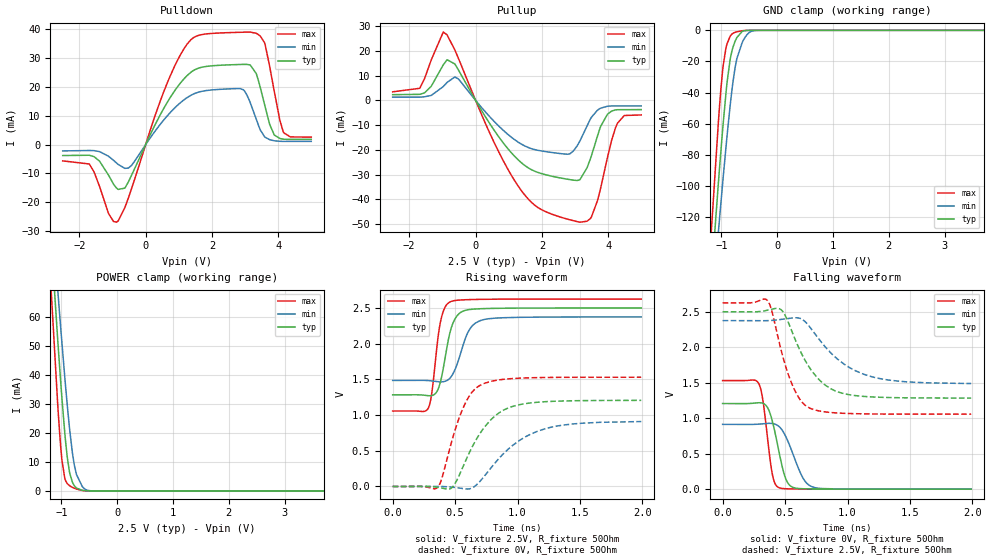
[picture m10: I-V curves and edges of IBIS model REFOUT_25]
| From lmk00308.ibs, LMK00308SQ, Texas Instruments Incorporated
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|   Model REFOUT_25
[Model]   REFOUT_25
Model_type   Output
Polarity   Non-Inverting
Rref =   50.0000
Vref =   1.25
Vmeas =   1.25
|   typ   min   max
C_comp   0.4681pF   0.4606pF   0.4681pF
|Output in low   Nom   Weak   Strong
|C_Comp   0.4681pF   0.4606pF   0.4681pF
|Output in High   Nom   Strong   Weak
|C_Comp High   0.4470pF   0.4470pF   0.4539pF
|Output in Hi-Z   Nom   Strong   Weak
|C_Comp   0.5714pF   0.5375pF   0.5943pF
[Voltage Range]   2.5   2.375   2.625
[Temperature Range]   45   125   -40
[Pullup Reference]   2.5   2.375   2.625
[Pulldown Reference]   0   0   0
[Power Clamp Reference]   2.5   2.375   2.625
[GND Clamp Reference]   0   0   0
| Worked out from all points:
|   slope of the pulldown table from 0 to 0.375 V, typ, clamps not added: 42 ohm
|   slope of the pullup table from 0 to 0.375 V, typ, clamps not added: 45.2 ohm
|   GND clamp passes 1 mA (typ) near -0.63 V on its own axis
|   POWER clamp passes 1 mA (typ) near -0.73 V on its own axis
|   falling waveform, V_fixture 0V, R_fixture 50Ohm: 20-80 % time 91.2ps typ, 127ps min, 64.1ps max; typ from 1.21 V to 0 V
|   rising waveform, V_fixture 2.5V, R_fixture 50Ohm: 20-80 % time 85.5ps typ, 110ps min, 65.7ps max; typ from 1.28 V to 2.5 V
|   rising waveform, V_fixture 0V, R_fixture 50Ohm: 20-80 % time 250ps typ, 348ps min, 176ps max; typ from 0 V to 1.21 V
|   falling waveform, V_fixture 2.5V, R_fixture 50Ohm: 20-80 % time 234ps typ, 332ps min, 163ps max; typ from 2.5 V to 1.28 V
[Pulldown]
|   Voltage   I(typ)   I(min)   I(max)
-2.5V     -3.786mA   -2.179mA   -5.641mA
-1.698V   -3.679mA   -2.038mA   -6.725mA
-1.12V    -10.57mA   -4.022mA   -23.89mA
-827.5mV  -15.55mA   -6.873mA   -26.48mA
-422.5mV  -10.57mA   -7.175mA   -15.18mA
890mV     18.94mA    12.9mA     27.64mA
1.895V    27.24mA    18.87mA    38.51mA
2.945V    27.86mA    19.05mA    39.03mA
3.455V    19.87mA    5.117mA    37.69mA
3.875V    3.399mA    1.343mA    18.61mA
4.145V    1.907mA    1.124mA    4.528mA
4.992V    1.816mA    1.12mA     2.598mA
[GND Clamp]
|   Voltage   I(typ)   I(min)   I(max)
-2.5V     -850.7mA   -783.9mA   -946.5mA
-1.202V   -170.8mA   -193.7mA   -141.7mA
-1.052V   -97.92mA   -129.5mA   -58.7mA
-1.038V   -90.97mA   -123.2mA   -51.32mA
-970mV    -61.13mA   -95.72mA   -23.37mA
-917.5mV  -40.48mA   -75.29mA   -11.35mA
-842.5mV  -18.81mA   -48.55mA   -3.881mA
-790mV    -10.67mA   -32.74mA   -1.863mA
-722.5mV  -4.664mA   -18.24mA   -948.5uA
-625mV    -674.1uA   -7.739mA   -269.5uA
-415mV    -2.631uA   -208.5uA   -1.695uA
4.992V    0A         0A         0A
[Pullup]
|   Voltage   I(typ)   I(min)   I(max)
-2.5V     2.292mA    1.299mA    3.442mA
-1.683V   2.418mA    1.287mA    4.854mA
-970mV    14.41mA    5.628mA    27.54mA
-520mV    12.32mA    8.65mA     17.02mA
537.5mV   -11.63mA   -8.192mA   -16.39mA
1.363V    -24.97mA   -17.52mA   -36.09mA
2.78V     -31.85mA   -21.73mA   -47.97mA
3.147V    -31.96mA   -16.32mA   -49.17mA
3.493V    -22.32mA   -6.811mA   -47.02mA
3.973V    -5.672mA   -2.384mA   -23.2mA
4.28V     -3.776mA   -2.257mA   -9.165mA
4.992V    -3.74mA    -2.236mA   -5.891mA
[POWER Clamp]
|   Voltage   I(typ)   I(min)   I(max)
-2.5V     504.8mA    460mA      565.3mA
-1.21V    94.23mA    106.3mA    77.92mA
-1.06V    50.38mA    67.9mA     27.85mA
-992.5mV  32.36mA    51.45mA    10.86mA
-940mV    20.01mA    39.28mA    4.347mA
-895mV    11.57mA    29.52mA    2.526mA
-850mV    6.048mA    20.73mA    1.745mA
-797.5mV  2.773mA    12.35mA    1.177mA
-730mV    975.1uA    5.644mA    633.8uA
-625mV    202.7uA    1.451mA    147.7uA
-490mV    13.53uA    84.98uA    8.561uA
4.992V    0A         0A         0A
[Ramp]
R_load = 50
|   typ   min   max
dV/dt_r   0.729929/8.55058e-11   0.533736/1.09569e-10   0.940882/6.56837e-11
dV/dt_f   0.723906/9.11659e-11   0.547724/1.26944e-10   0.918161/6.41243e-11
[Falling Waveform]
V_fixture = 0V
V_fixture_min = 0V
V_fixture_max = 0V
R_fixture = 50Ohm
C_fixture = 0F
|   Time   V(typ)   V(min)   V(max)
0s        1.207V     912.9mV    1.53V
290ps     1.218V     916.5mV    1.486V
325ps     1.208V     921.6mV    1.223V
400ps     946.1mV    924.1mV    194.5mV
450ps     539mV      885.5mV    21.86mV
495ps     200.8mV    778.8mV    7.086mV
535ps     58.33mV    623.1mV    4.333mV
645ps     5.891mV    152.6mV    1.862mV
735ps     2.902mV    23.04mV    1.029mV
1.99ns    3.135uV    31.66uV    361nV
[Rising Waveform]
V_fixture = 2.5V
V_fixture_min = 2.375V
V_fixture_max = 2.625V
R_fixture = 50Ohm
C_fixture = 0F
|   Time   V(typ)   V(min)   V(max)
0s        1.283V     1.485V     1.057V
285ps     1.272V     1.483V     1.096V
315ps     1.275V     1.478V     1.33V
360ps     1.348V     1.468V     2.044V
385ps     1.483V     1.466V     2.323V
460ps     2.163V     1.52V      2.585V
520ps     2.399V     1.733V     2.609V
605ps     2.476V     2.167V     2.617V
710ps     2.49V      2.328V     2.621V
1.99ns    2.5V       2.375V     2.625V
[Rising Waveform]
V_fixture = 0V
V_fixture_min = 0V
V_fixture_max = 0V
R_fixture = 50Ohm
C_fixture = 0F
|   Time   V(typ)   V(min)   V(max)
0s        4.384nV    8.988nV    3.562nV
365ps     -12.65mV   610.3uV    -4.348mV
470ps     -23.12mV   -8.83mV    613.4mV
560ps     263.3mV    -28.69mV   1.083V
635ps     547.9mV    -21.33mV   1.319V
720ps     795.7mV    114.2mV    1.434V
900ps     1.08V      481.4mV    1.503V
1.165ns   1.18V      776.7mV    1.525V
1.445ns   1.201V     876.2mV    1.529V
1.99ns    1.206V     909.3mV    1.53V
[Falling Waveform]
|Gnd
V_fixture = 2.5V
V_fixture_min = 2.375V
V_fixture_max = 2.625V
R_fixture = 50Ohm
C_fixture = 0F
|   Time   V(typ)   V(min)   V(max)
0s        2.5V       2.375V     2.625V
360ps     2.522V     2.375V     2.657V
390ps     2.534V     2.378V     2.537V
470ps     2.526V     2.392V     1.949V
545ps     2.267V     2.409V     1.526V
620ps     1.954V     2.406V     1.263V
700ps     1.702V     2.281V     1.141V
870ps     1.412V     1.914V     1.08V
1.135ns   1.306V     1.617V     1.061V
1.99ns    1.284V     1.488V     1.057V
